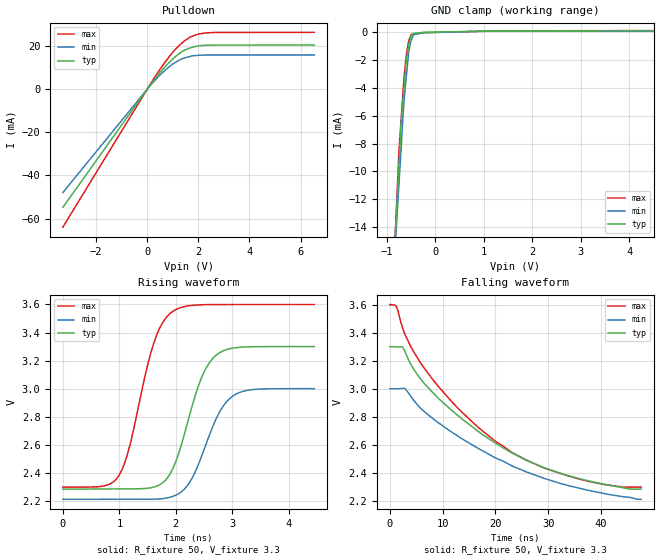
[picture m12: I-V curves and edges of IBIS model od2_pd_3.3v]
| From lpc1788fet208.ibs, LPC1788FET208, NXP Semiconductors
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[Model]   od2_pd_3.3v
Model_type I/O_open_drain
Vinl=9.900E-01
Vinh=2.310E+00
Vref=3.300E+00
Rref=2.000E+03
Cref=0.000E+00
Vmeas=1.650E+00
C_comp   5.160E-13   4.910E-13   5.420E-13
[Voltage Range]   3.300E+00   3.000E+00   3.600E+00
[POWER Clamp Reference]   3.300E+00   3.000E+00   3.600E+00
[GND Clamp Reference]   0.000E+00   0.000E+00   0.000E+00
[Pullup Reference]   3.300E+00   3.000E+00   3.600E+00
[Pulldown Reference]   0.000E+00   0.000E+00   0.000E+00
[Temperature Range]   25   85   -40
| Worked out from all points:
|   slope of the pulldown table from 0 to 0.495 V, typ, clamps not added: 64.9 ohm
|   GND clamp passes 1 mA (typ) near -0.55 V on its own axis
|   rising waveform, R_fixture 50, V_fixture 3.3: 20-80 % time 470ps typ, 490ps min, 462ps max; typ from 2.28 V to 3.3 V
|   falling waveform, R_fixture 50, V_fixture 3.3: 20-80 % time 20.8ns typ, 22.3ns min, 19.2ns max; typ from 3.3 V to 2.28 V
[GND Clamp]
-3.3V     -177.3mA   -158.8mA   -207.6mA
-750mV    -9.48mA    -10.87mA   -8.485mA
-700mV    -6.189mA   -7.965mA   -5.957mA
-650mV    -4.159mA   -5.063mA   -3.43mA
-600mV    -2.128mA   -3.252mA   -1.687mA
-550mV    -914.7uA   -1.441mA   -630.3uA
-500mV    -306.1uA   -590.9uA   -184.3uA
-450mV    -93.32uA   -195.9uA   -156.7uA
-225mV    -19.98uA   -51.54uA   -44.27uA
1.05V     62.05uA    54.96uA    59.19uA
6.6V      98.62uA    85.9uA     109.4uA
[Pulldown]
-3.3V     -54.79mA   -47.91mA   -63.96mA
153mV     2.489mA    2.147mA    2.94mA
512.3mV   7.874mA    6.706mA    9.412mA
891.5mV   12.77mA    10.7mA     15.54mA
1.131V    15.41mA    12.66mA    18.82mA
1.43V     17.91mA    14.39mA    22.12mA
1.77V     19.45mA    15.47mA    24.58mA
2.269V    20.35mA    15.84mA    26.06mA
6.54V     20.51mA    15.9mA     26.38mA
[Rising Waveform]
R_fixture = 50
V_fixture = 3.3
V_fixture_min = 3
V_fixture_max = 3.6
0s        2.284V     2.211V     2.298V
1ns       2.285V     2.212V     2.386V
1.2ns     2.286V     2.212V     2.619V
1.6ns     2.297V     2.212V     3.314V
1.95ns    2.433V     2.233V     3.552V
2.3ns     2.893V     2.372V     3.594V
2.5ns     3.12V      2.567V     3.598V
2.7ns     3.234V     2.774V     3.6V
3.15ns    3.295V     2.976V     3.6V
4.45ns    3.3V       3V         3.6V
[Falling Waveform]
R_fixture = 50
V_fixture = 3.3
V_fixture_min = 3
V_fixture_max = 3.6
0s        3.3V       3V         3.6V
1.199ns   3.299V     3V         3.589V
2.447ns   3.295V     3.003V     3.433V
5.194ns   3.102V     2.888V     3.223V
8.241ns   2.969V     2.785V     3.061V
13.99ns   2.776V     2.636V     2.822V
20.13ns   2.609V     2.504V     2.622V
25.82ns   2.491V     2.407V     2.491V
32.62ns   2.394V     2.321V     2.392V
47.6ns    2.284V     2.211V     2.298V
[Ramp]
dV/dt_r   6.0988E-01/4.6880E-10   4.7340E-01/4.8990E-10   7.8133E-01/4.6000E-10
dV/dt_f   6.0988E-01/2.0795E-08   4.7340E-01/2.2268E-08   7.8133E-01/1.9147E-08
R_load = 50
